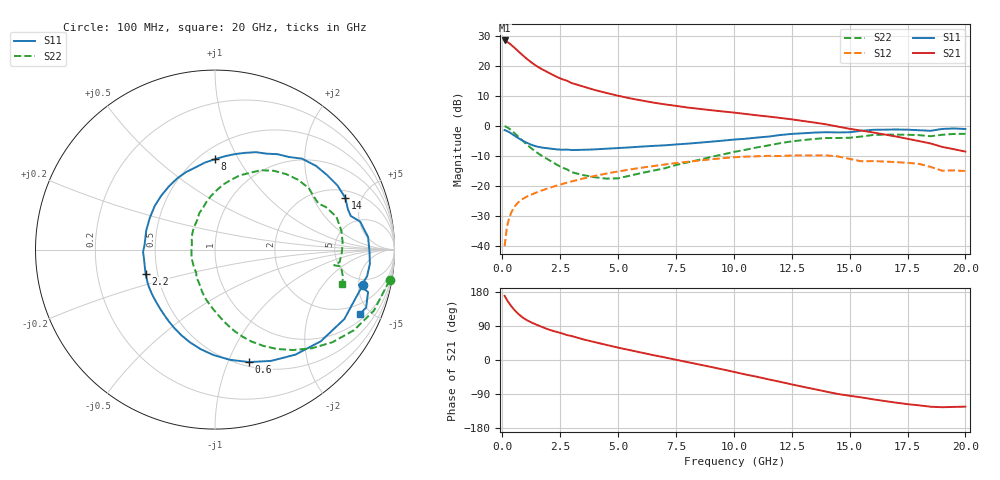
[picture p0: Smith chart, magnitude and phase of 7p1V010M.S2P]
! Infineon Technologies  Discrete & RF Semiconductors
! bfp620
! VCE =  1.0 V,  IC =  10 mA
! Common Emitter S-Parameters:  Sep 2002
# GHz  S  MA  R  50
!  f  S11  S21  S12  S22
! GHz  MAG  ANG  MAG  ANG  MAG  ANG  MAG  ANG
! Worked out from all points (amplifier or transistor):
!   59 points, 100 MHz to 20 GHz, reference 50 ohm
!   highest |S21| = 28.5 dB at 100 MHz (marker M1)
!   |S21| within 3 dB of that: start of sweep to 605.4 MHz
!   unconditionally stable (mu >= 1): 4.143 GHz to 10.52 GHz; 17.04 GHz to end of sweep
!   at 1 GHz: K = 0.50, MSG = 23.3 dB, |S12| = -23.9 dB
!   at 5.5 GHz: K = 1.04, MAG = 10.6 dB, |S12| = -14.6 dB
!   at 20 GHz: K = 1.44, MAG = -0.7 dB, |S12| = -15.1 dB
!   S11 on the Smith chart (normalised r, x): 100 MHz: 4.07, -5.64; 600 MHz: 0.54, -1.20; 2.2 GHz: 0.43, -0.14; 8 GHz: 0.59, +0.80; 14 GHz: 2.46, +3.64; 20 GHz: 1.32, -4.32
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0.1  0.8467 -13.4  26.51 169.3  0.0098 81.5  0.9874 -10.0
0.2  0.818 -28.2  25.29 158.5  0.0204 76.0  0.9484 -21.0
0.3  0.7801 -40.9  23.78 149.3  0.0292 70.4  0.8951 -30.1
0.4  0.7373 -52.5  22.12 141.1  0.0366 65.3  0.8339 -38.2
0.5  0.6946 -63.2  20.45 133.8  0.0429 61.0  0.7706 -45.5
0.6  0.655 -73.1  18.85 127.2  0.0484 57.4  0.7092 -52.1
0.7  0.6195 -82.3  17.37 121.2  0.0531 54.4  0.652 -58.1
0.9  0.56 -98.3  14.79 111.4  0.0607 50.0  0.5525 -68.2
1  0.5349 -105.2  13.7 107.4  0.0639 48.4  0.51 -72.3
1.2  0.4926 -117.3  11.86 100.8  0.0696 46.1  0.4381 -79.3
1.7  0.4341 -141.5  8.846 87.5  0.083 42.7  0.3174 -93.9
2.2  0.4102 -160.4  7.015 76.6  0.0964 40.1  0.2433 -107.4
3  0.3933 175.9  5.152 63.2  0.118 35.5  0.168 -128.2
3.5  0.3975 164.6  4.51 54.4  0.1322 32.2  0.1502 -142.6
5  0.4247 134.6  3.171 32.7  0.1731 20.8  0.1328 166.0
7  0.4713 103.1  2.282 7.1  0.2255 3.6  0.1946 120.1
8  0.5032 90.2  2.016 -5.6  0.2502 -6.2  0.2447 105.4
10.5  0.607 61.7  1.575 -38.2  0.3055 -33.7  0.3975 77.2
13.5  0.7701 27.7  1.128 -77.1  0.3195 -67.5  0.604 40.2
14  0.7811 21.7  1.054 -83.6  0.3202 -74.1  0.6247 33.3
17  0.8666 -5.3  0.663 -112.5  0.2474 -98.3  0.7122 3.4
20  0.8831 -24.0  0.371 -123.1  0.1757 -110.1  0.7337 -15.2
